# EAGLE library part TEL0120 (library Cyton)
IC: SoC; GPIO, I2C, I2S, IR, SD, SDIO, SPI, UART; 2.7÷3.6VDC; 20dBm
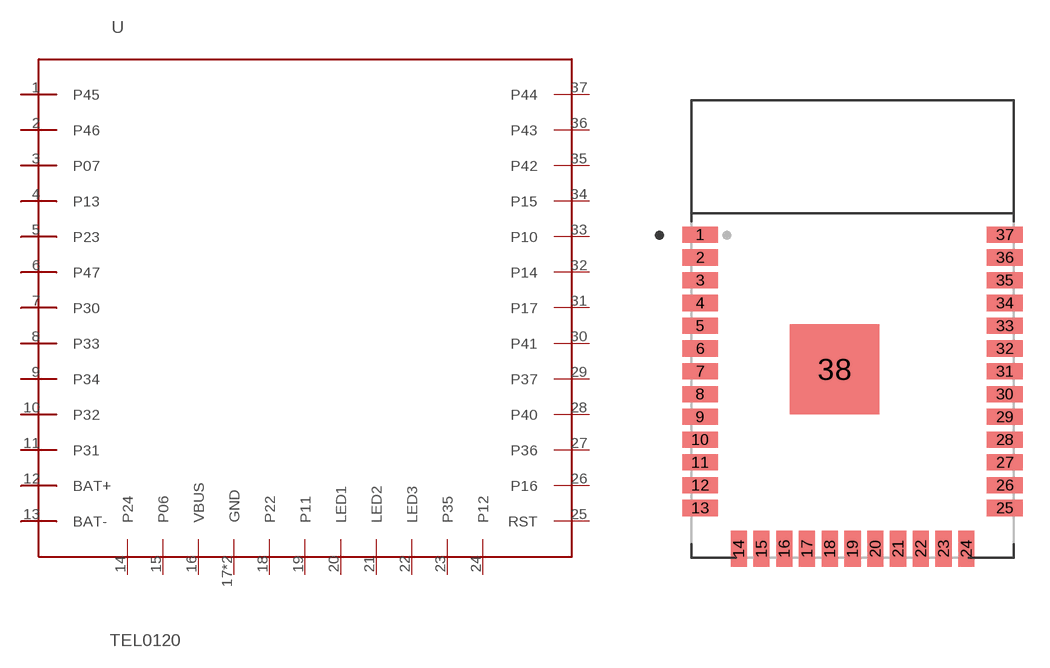
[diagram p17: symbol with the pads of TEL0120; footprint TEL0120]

Designator prefix U

## TEL0120 (AVAILABILITY: Unavailable; DESCRIPTION: IC: SoC; GPIO, I2C, I2S, IR, SD, SDIO, SPI, UART; 2.7÷3.6VDC; 20dBm; MF: Espressif Systems; MP: ESP32-WROOM-32D; PACKAGE: Module Espressif Systems; PRICE: None)  [TEL0120]
1  P45
2  P46
3  P07
4  P13
5  P23
6  P47
7  P30
8  P33
9  P34
10  P32
11  P31
12  BAT+
13  BAT-
14  P24
15  P06
16  VBUS
17  GND
18  P22
19  P11
20  LED1
21  LED2
22  LED3
23  P35
24  P12
25  RST
26  P16
27  P36
28  P40
29  P37
30  P41
31  P17
32  P14
33  P10
34  P15
35  P42
36  P43
37  P44
38  GND

## Footprint TEL0120 (pad centres in mm)
smd 2 x 0.9: 1 -8.5,5.26; 2 -8.5,3.99; 3 -8.5,2.72; 4 -8.5,1.45; 5 -8.5,0.18; 6 -8.5,-1.09; 7 -8.5,-2.36; 8 -8.5,-3.63; 9 -8.5,-4.9; 10 -8.5,-6.17; 11 -8.5,-7.44; 12 -8.5,-8.71; 13 -8.5,-9.98; 25 8.5,-9.98; 26 8.5,-8.71; 27 8.5,-7.44; 28 8.5,-6.17; 29 8.5,-4.9; 30 8.5,-3.63; 31 8.5,-2.36; 32 8.5,-1.09; 33 8.5,0.18; 34 8.5,1.45; 35 8.5,2.72; 36 8.5,3.99; 37 8.5,5.26
smd 0.9 x 2: 14 -6.35,-12.25; 15 -5.08,-12.25; 16 -3.81,-12.25; 17 -2.54,-12.25; 18 -1.27,-12.25; 19 0,-12.25; 20 1.27,-12.25; 21 2.54,-12.25; 22 3.81,-12.25; 23 5.08,-12.25; 24 6.35,-12.25
smd 5 x 5: 38 -1,-2.24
